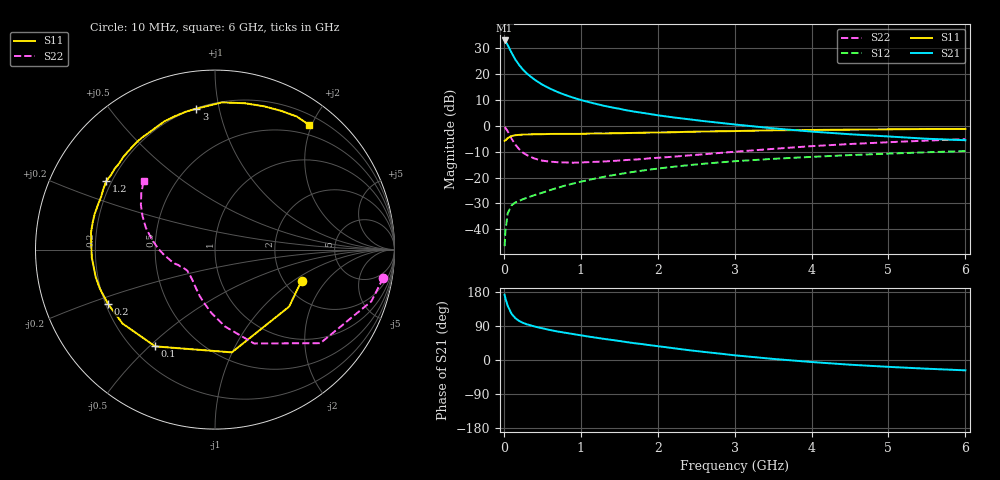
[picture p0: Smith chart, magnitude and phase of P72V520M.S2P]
! SIEMENS Small Signal Semiconductors
! BFP196
! Si NPN RF Bipolar Junction Transistor in SOT143
! VCE = 2.5 V  IC = 20 mA
! Common Emitter S-Parameters:  May  1996
# GHz  S  MA  R  50
!  f  S11  S21  S12  S22
! GHz  MAG  ANG  MAG  ANG  MAG  ANG  MAG  ANG
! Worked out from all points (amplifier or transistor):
!   36 points, 10 MHz to 6 GHz, reference 50 ohm
!   highest |S21| = 33.0 dB at 10 MHz (marker M1)
!   |S21| within 3 dB of that: start of sweep to 71.03 MHz
!   unconditionally stable (mu >= 1): 665.2 MHz to 3.418 GHz; 3.899 GHz to 4.059 GHz
!   at 250 MHz: K = 0.61, MSG = 25.0 dB, |S12| = -28.4 dB
!   at 1.4 GHz: K = 1.12, MAG = 11.1 dB, |S12| = -19.2 dB
!   at 6 GHz: K = 0.96, MSG = 2.1 dB, |S12| = -9.7 dB
!   S11 on the Smith chart (normalised r, x): 10 MHz: 2.47, -1.17; 100 MHz: 0.29, -0.52; 200 MHz: 0.21, -0.23; 1.2 GHz: 0.18, +0.28; 3 GHz: 0.20, +0.86; 6 GHz: 0.34, +1.96
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0.01  0.5131 -19.9  44.89 172.2  0.0047 82.5  0.9502 -9.6
0.02  0.5208 -37.7  43.11 163.1  0.0091 76.7  0.9177 -18.3
0.05  0.5802 -80.7  36.73 143.2  0.0202 59.6  0.7852 -41.6
0.1  0.6338 -121.7  26.04 122.0  0.0289 45.9  0.5665 -67.4
0.15  0.6596 -141.3  19.12 110.3  0.033 40.8  0.432 -82.6
0.2  0.6689 -153.3  15 103.0  0.0354 40.1  0.3528 -93.4
0.25  0.6773 -161.4  12.15 97.9  0.0382 40.5  0.3012 -102.0
0.3  0.6821 -167.1  10.26 94.1  0.0406 42.2  0.2716 -108.4
0.4  0.6878 -176.2  7.812 88.4  0.0458 45.0  0.2323 -118.5
0.5  0.6899 177.9  6.269 83.7  0.0509 47.4  0.2122 -126.1
0.6  0.6975 172.1  5.248 79.2  0.0571 49.8  0.2029 -131.7
0.7  0.698 167.3  4.508 75.2  0.0634 51.1  0.198 -135.9
0.9  0.6982 159.0  3.515 68.5  0.0765 52.4  0.1936 -142.3
1.1  0.7073 151.7  2.891 61.9  0.0897 52.9  0.1987 -146.8
1.2  0.7161 147.7  2.658 58.8  0.0966 52.7  0.2016 -149.0
1.6  0.7262 134.8  1.995 47.1  0.1231 50.2  0.2187 -155.7
2.2  0.7518 117.5  1.458 31.3  0.1614 44.0  0.2528 -165.5
3  0.7921 97.5  1.064 12.4  0.2068 34.1  0.3152 179.4
3.5  0.8209 87.3  0.896 2.9  0.23 28.0  0.3585 170.4
4.5  0.8441 71.0  0.688 -12.4  0.2717 16.6  0.445 155.2
5.5  0.8701 58.5  0.563 -23.0  0.3084 5.7  0.5188 142.3
6  0.8707 53.0  0.527 -27.3  0.3255 -0.1  0.5514 136.1
